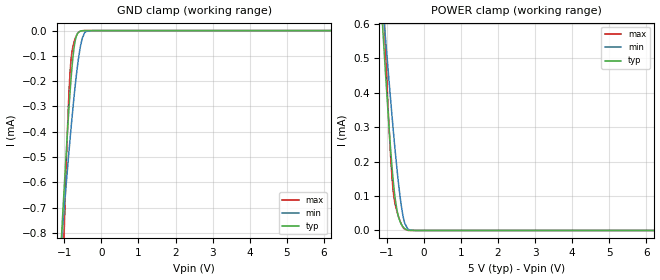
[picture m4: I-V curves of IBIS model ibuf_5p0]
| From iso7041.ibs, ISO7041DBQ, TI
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|   ibuf_5p0 Model
[Model]   ibuf_5p0
Model_type   Input
Vinl = 1.5
Vinh = 3.5
|   typ   min   max
C_comp   0.001pF   0.001pF   0.020pF
[Model spec]
|subparameter
Vinl   1.5   1.35   1.65
Vinh   3.5   3.15   3.85
| Where Nom  PVT is Nominal Process, 5.0V, 27C
|   Fast PVT is Strong Process,  5.5V, -55C
|   Slow PVT is Weak Process,   4.5V, 150C
[Voltage Range]   5   4.5   5.5
|Junction Temperature
[Temperature Range]   27   150   -55
[Power Clamp Reference]   5   4.5   5.5
[GND Clamp Reference]   0   0   0
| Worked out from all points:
|   GND clamp passes 1 mA (typ) near -1.14 V on its own axis
[GND Clamp]
|   Voltage   I(typ)   I(min)   I(max)
-5V       -12.37mA   -8.463mA   -24.93mA
-1.07V    -798uA     -821.3uA   -1.134mA
-1.04V    -718uA     -767.3uA   -978.5uA
-1.01V    -639.2uA   -713.7uA   -827.1uA
-890mV    -341.9uA   -504.8uA   -297.3uA
-830mV    -212.9uA   -405uA     -135uA
-785mV    -132.4uA   -333.3uA   -76.39uA
-710mV    -43.31uA   -222.9uA   -32.78uA
-560mV    -1.879uA   -58.23uA   -1.792uA
-440mV    -79.87nA   -6.647uA   -34.52nA
-230mV    0A         -17.98nA   0A
10V       0A         0A         0A
[POWER Clamp]
|   Voltage   I(typ)   I(min)   I(max)
-5V       89.69mA    35.2mA     146.1mA
-1.13V    621.9uA    685.1uA    772.5uA
-1.04V    464.5uA    564.6uA    533.3uA
-950mV    315.6uA    446.7uA    321.6uA
-905mV    246.9uA    389.2uA    229.5uA
-860mV    184.5uA    333uA      154.5uA
-815mV    131.3uA    278.5uA    103uA
-725mV    58.69uA    177.3uA    54.61uA
-605mV    17.52uA    69.14uA    17.5uA
-530mV    6.361uA    26.37uA    4.889uA
-440mV    1.058uA    5.186uA    483nA
10V       0A         0A         0A
